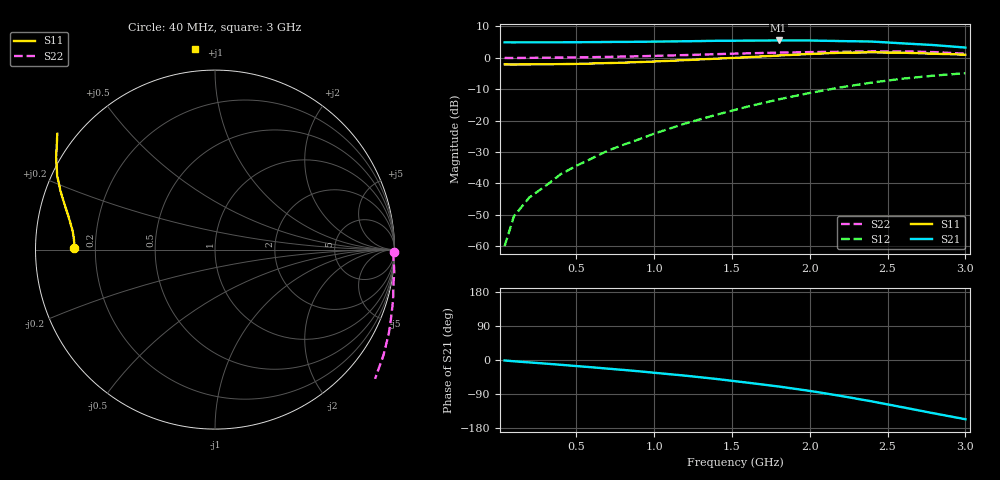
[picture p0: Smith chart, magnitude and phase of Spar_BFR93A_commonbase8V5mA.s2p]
! Filename:  BFR93ACE.S2P  Version:  2.0
! NXP part #: BFR93A  Date: Jul 1990
! Bias condition: Vce=8V, Ic=5mA
! COMMON BASE
#  MHz  S  MA  R  50
! Freq  S11  S21  S12  S22
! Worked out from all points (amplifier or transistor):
!   21 points, 40 MHz to 3 GHz, reference 50 ohm
!   highest |S21| = 5.5 dB at 1.8 GHz (marker M1)
!   |S21| within 3 dB of that: start of sweep to end of sweep
!   unconditionally stable (mu >= 1): start of sweep to 47.2 MHz
!   at 300 MHz: K = -0.51, MSG = 22.9 dB, |S12| = -40.9 dB
!   at 1 GHz: K = -0.89, MSG = 14.7 dB, |S12| = -24.2 dB
!   at 3 GHz: K = -0.46, MSG = 4.1 dB, |S12| = -4.9 dB
40  0.785 179.3  1.767 -1.2  0.001 59.0  0.996 -0.8
100  0.784 178.1  1.766 -3.4  0.003 90.8  0.995 -2.6
200  0.786 176.7  1.769 -6.4  0.006 100.6  1 -4.7
300  0.79 175.2  1.768 -9.4  0.009 113.3  1.007 -7.2
400  0.795 173.7  1.768 -12.6  0.014 119.3  1.01 -9.7
500  0.802 172.2  1.776 -16.0  0.019 125.5  1.017 -12.3
600  0.813 170.5  1.781 -19.2  0.025 129.3  1.027 -14.8
700  0.825 168.8  1.791 -22.7  0.033 131.6  1.037 -17.5
800  0.839 167.0  1.795 -26.1  0.041 134.6  1.048 -20.3
900  0.856 165.2  1.804 -29.7  0.05 136.3  1.061 -23.0
1000  0.875 163.3  1.816 -33.6  0.062 137.0  1.076 -25.9
1200  0.92 159.3  1.837 -41.3  0.09 137.8  1.108 -32.1
1400  0.971 154.9  1.87 -50.0  0.124 136.1  1.146 -38.9
1600  1.024 149.8  1.883 -59.8  0.167 134.1  1.182 -46.3
1800  1.09 143.7  1.894 -69.9  0.218 129.7  1.212 -54.7
2000  1.153 137.1  1.892 -81.5  0.276 124.4  1.235 -64.3
2200  1.207 130.3  1.851 -94.8  0.339 118.1  1.251 -75.6
2400  1.224 122.5  1.819 -109.3  0.404 110.4  1.271 -87.5
2600  1.208 114.0  1.7 -125.0  0.467 102.4  1.269 -98.8
2800  1.164 104.6  1.597 -140.9  0.522 94.0  1.234 -109.9
3000  1.124 95.7  1.459 -156.3  0.57 86.9  1.165 -120.3
